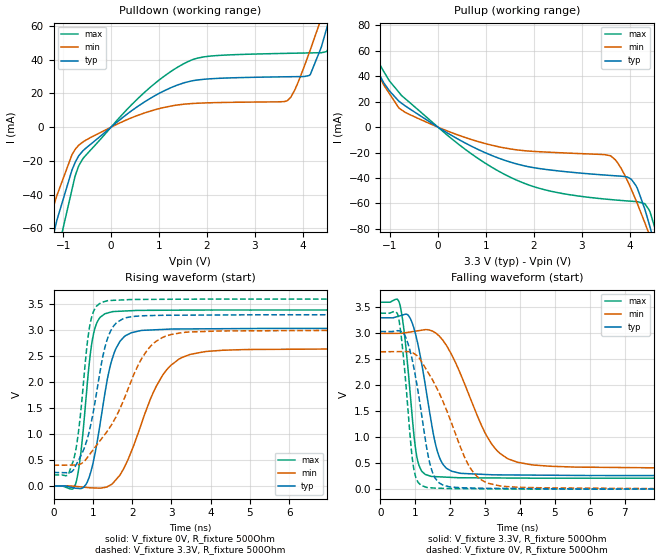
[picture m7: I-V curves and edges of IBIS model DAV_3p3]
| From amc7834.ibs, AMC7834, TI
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|   Model
[Model]   DAV_3p3
Model_type   Output
Polarity   Non-Inverting
Vmeas = 1.65
Vref = 0
Cref = 1pF
Rref = 100000
|   typ   min   max
C_comp   3.504pF   3.144pF   3.899pF
[Voltage Range]   3.3   3   3.6
[Temperature Range]   27   125   -40
[Pullup Reference]   3.3   3   3.6
[Pulldown Reference]   0   0   0
[Power Clamp Reference]   3.3   3   3.6
[GND Clamp Reference]   0   0   0
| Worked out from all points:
|   slope of the pulldown table from 0 to 0.495 V, typ, clamps not added: 44.7 ohm
|   slope of the pullup table from 0 to 0.495 V, typ, clamps not added: 45 ohm
|   falling waveform, V_fixture 3.3V, R_fixture 500Ohm: 20-80 % time 474ps typ, 1.02ns min, 287ps max; typ from 3.3 V to 0.259 V
|   rising waveform, V_fixture 0V, R_fixture 500Ohm: 20-80 % time 434ps typ, 857ps min, 266ps max; typ from 0 V to 3.04 V
|   rising waveform, V_fixture 3.3V, R_fixture 500Ohm: 20-80 % time 472ps typ, 1.03ns min, 281ps max; typ from 0.259 V to 3.3 V
|   falling waveform, V_fixture 0V, R_fixture 500Ohm: 20-80 % time 449ps typ, 991ps min, 264ps max; typ from 3.04 V to 0 V
[Pulldown]
|   Voltage   I(typ)   I(min)   I(max)
-3.3V     -391.3mA   -286.7mA   -484.8mA
-1.421V   -94.52mA   -68.84mA   -120mA
-1.132V   -55.39mA   -40.72mA   -76.18mA
-587.4mV  -14.04mA   -8.793mA   -18.71mA
699.6mV   15.01mA    8.431mA    20.7mA
1.67V     27.34mA    13.96mA    39.69mA
3.679V    29.87mA    15.78mA    43.76mA
4.155V    31.18mA    45.85mA    44.01mA
4.382V    47.3mA     64.44mA    44.14mA
4.491V    58.06mA    73.55mA    44.79mA
4.907V    102mA      107.3mA    81.35mA
6.6V      236.8mA    205.6mA    261mA
[Pullup]
|   Voltage   I(typ)   I(min)   I(max)
-3.3V     208.9mA    178.4mA    240.2mA
-1.983V   115.9mA    100.6mA    133.2mA
-1.32V    51.36mA    47.92mA    57.3mA
-1.132V   34.96mA    33.29mA    43.87mA
-815.1mV  20.38mA    15.03mA    27.45mA
590.7mV   -12.94mA   -8.442mA   -18.08mA
1.67V     -29.24mA   -18mA      -42.19mA
3.61V     -38.05mA   -22.81mA   -57.03mA
4.036V    -41.22mA   -49.24mA   -58.32mA
4.402V    -75.88mA   -84.03mA   -65.02mA
4.788V    -131mA     -125mA     -112.4mA
6.6V      -419.6mA   -342.1mA   -462.8mA
[Ramp]
R_load = 500
|   typ   min   max
dV/dt_r   1.82193/4.33867e-10   1.58773/8.55982e-10   2.03399/2.65634e-10
dV/dt_f   1.82452/4.7376e-10   1.5617/1.01925e-09   2.0337/2.86631e-10
[Falling Waveform]
V_fixture = 3.3V
V_fixture_min = 3V
V_fixture_max = 3.6V
R_fixture = 500Ohm
C_fixture = 0F
|   Time   V(typ)   V(min)   V(max)
0s        3.3V       3V         3.6V
565.6ps   3.34V      3.001V     3.536V
789.6ps   3.356V     3.021V     2.324V
1.036ns   2.907V     3.046V     657.1mV
1.46ns    1.285V     3.053V     245.2mV
1.692ns   612.9mV    2.945V     237.5mV
2.045ns   345.4mV    2.587V     226.2mV
3.193ns   277.4mV    865.7mV    216.3mV
4.306ns   270.9mV    472mV      212mV
30ns      259.1mV    397.2mV    210.5mV
[Rising Waveform]
V_fixture = 0V
V_fixture_min = 0V
V_fixture_max = 0V
R_fixture = 500Ohm
C_fixture = 0F
|   Time   V(typ)   V(min)   V(max)
0s        1.643uV    -18.33uV   113.5nV
565.6ps   -45.6mV    -9.505mV   46.81mV
693.3ps   -51.47mV   -19.17mV   621.7mV
854.1ps   65.89mV    -31.34mV   1.922V
1.088ns   751.9mV    -41.26mV   3.115V
1.497ns   2.454V     38.43mV    3.357V
1.835ns   2.896V     410.2mV    3.371V
2.776ns   3.015V     2.13V      3.385V
3.856ns   3.027V     2.587V     3.389V
30ns      3.037V     2.646V     3.39V
[Rising Waveform]
V_fixture = 3.3V
V_fixture_min = 3V
V_fixture_max = 3.6V
R_fixture = 500Ohm
C_fixture = 0F
|   Time   V(typ)   V(min)   V(max)
0s        259.1mV    397.2mV    210.5mV
492.7ps   295.7mV    401.3mV    459.7mV
651ps     516.3mV    414.1mV    1.136V
789.6ps   742.6mV    481.1mV    2.221V
895.6ps   1.008V     584mV      2.961V
1.017ns   1.444V     704.2mV    3.358V
1.381ns   2.852V     1.068V     3.57V
2.398ns   3.281V     2.628V     3.594V
3.344ns   3.29V      2.959V     3.597V
30ns      3.3V       3V         3.6V
[Falling Waveform]
|Gnd
V_fixture = 0V
V_fixture_min = 0V
V_fixture_max = 0V
R_fixture = 500Ohm
C_fixture = 0F
|   Time   V(typ)   V(min)   V(max)
0s        3.037V     2.646V     3.39V
511.8ps   3.051V     2.648V     3.329V
719.2ps   2.936V     2.649V     2.111V
950.8ps   2.364V     2.617V     417.4mV
1.071ns   1.912V     2.558V     141.3mV
1.327ns   797.5mV    2.292V     33.95mV
1.65ns    142mV      1.899V     17.89mV
2.612ns   22.23mV    370.4mV    8.2mV
3.479ns   14.52mV    58.23mV    4.762mV
30ns      -6.111uV   -60.63uV   621.3nV
